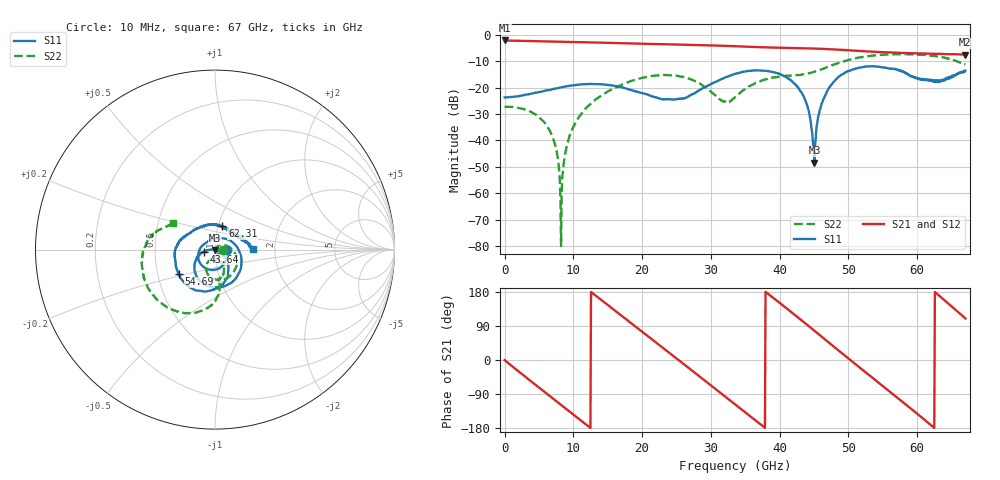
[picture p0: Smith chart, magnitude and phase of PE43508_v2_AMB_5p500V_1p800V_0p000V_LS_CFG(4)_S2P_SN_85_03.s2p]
!Keysight Technologies,N5227A,US51270237,A.10.43.00
!Date: Wednesday, August 22, 2018 17:06:55
!Correction: S11(Full 2 Port(1,3))
!S31(Full 2 Port(1,3))
!S13(Full 2 Port(1,3))
!S33(Full 2 Port(1,3))
!S2P File: Measurements: S11, S31, S13, S33:
# Hz S  dB  R 50
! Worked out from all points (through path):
!   801 points, 10 MHz to 67 GHz, reference 50 ohm
!   highest |S21| = -2.17 dB at 10 MHz (marker M1); lowest = -7.5 dB at 66.92 GHz (marker M2)
!   group delay of S21, straight-line fit = 39.9 ps
!   lowest |S11| = -48.4 dB at 45.06 GHz (marker M3), VSWR 1.01, Z = 50.1 - j0.365 ohm
!   |S11| at or under -10 dB: start of sweep to end of sweep
!   |S22| runs from -80.1 to -7.3 dB; largest |S21 - S12| = 0.0054
!   S11 on the Smith chart (normalised r, x): 10 MHz: 1.14, -0.00; 43.64 GHz: 0.89, -0.02; 54.69 GHz: 0.64, -0.19; 62.31 GHz: 1.05, +0.28; 67 GHz: 1.53, +0.01
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1e7  -23.71 -0.6  -2.17 -0.2  -2.17 -0.2  -27.24 -1.4
6.0391e9  -21.14 -45.7  -2.51 -87.6  -2.51 -87.5  -34.07 -75.2
7.3789e9  -20.38 -58.7  -2.59 -106.7  -2.59 -106.7  -41.97 -92.6
8.216275e9  -19.95 -67.2  -2.64 -118.6  -2.64 -118.6  -80.09 46.4
9.304862e9  -19.40 -77.8  -2.71 -134.1  -2.71 -134.1  -39.51 62.6
1.123082e10  -18.80 -97.8  -2.83 -161.4  -2.83 -161.4  -29.78 44.2
1.734366e10  -20.09 -162.7  -3.23 112.2  -3.21 112.2  -18.61 -13.3
2.236791e10  -24.01 143.7  -3.55 41.4  -3.54 41.3  -15.37 -62.8
2.697348e10  -23.02 64.9  -3.83 -23.8  -3.82 -23.9  -16.78 -105.4
3.032298e10  -18.27 7.9  -4.08 -71.7  -4.07 -71.7  -22.30 -119.4
3.3505e10  -14.86 -39.1  -4.35 -117.2  -4.35 -117.1  -23.73 -69.6
3.836178e10  -13.83 -103.5  -4.82 173.9  -4.81 174.0  -16.66 -72.9
4.363724e10  -24.26 -169.6  -5.12 98.1  -5.12 98.1  -14.93 -82.7
4.472582e10  -36.98 -179.7  -5.20 82.0  -5.19 82.1  -14.27 -82.7
4.506078e10  -48.42 -74.0  -5.24 77.0  -5.22 77.1  -14.03 -82.9
4.606562e10  -26.39 -30.5  -5.33 62.2  -5.31 62.0  -13.17 -83.6
4.790785e10  -17.74 -55.1  -5.55 34.7  -5.55 34.7  -11.28 -88.4
5.469059e10  -12.27 -145.5  -6.55 -64.1  -6.53 -64.4  -7.63 -128.7
5.586291e10  -12.83 -163.3  -6.69 -81.2  -6.68 -81.6  -7.43 -136.4
6.23107e10  -17.17 72.8  -7.22 -176.7  -7.26 -176.9  -8.01 -179.0
6.691626e10  -14.00 3.0  -7.53 111.0  -7.59 111.2  -11.19 149.2
6.7e10  -13.53 0.9  -7.52 109.6  -7.58 109.9  -11.26 147.8
